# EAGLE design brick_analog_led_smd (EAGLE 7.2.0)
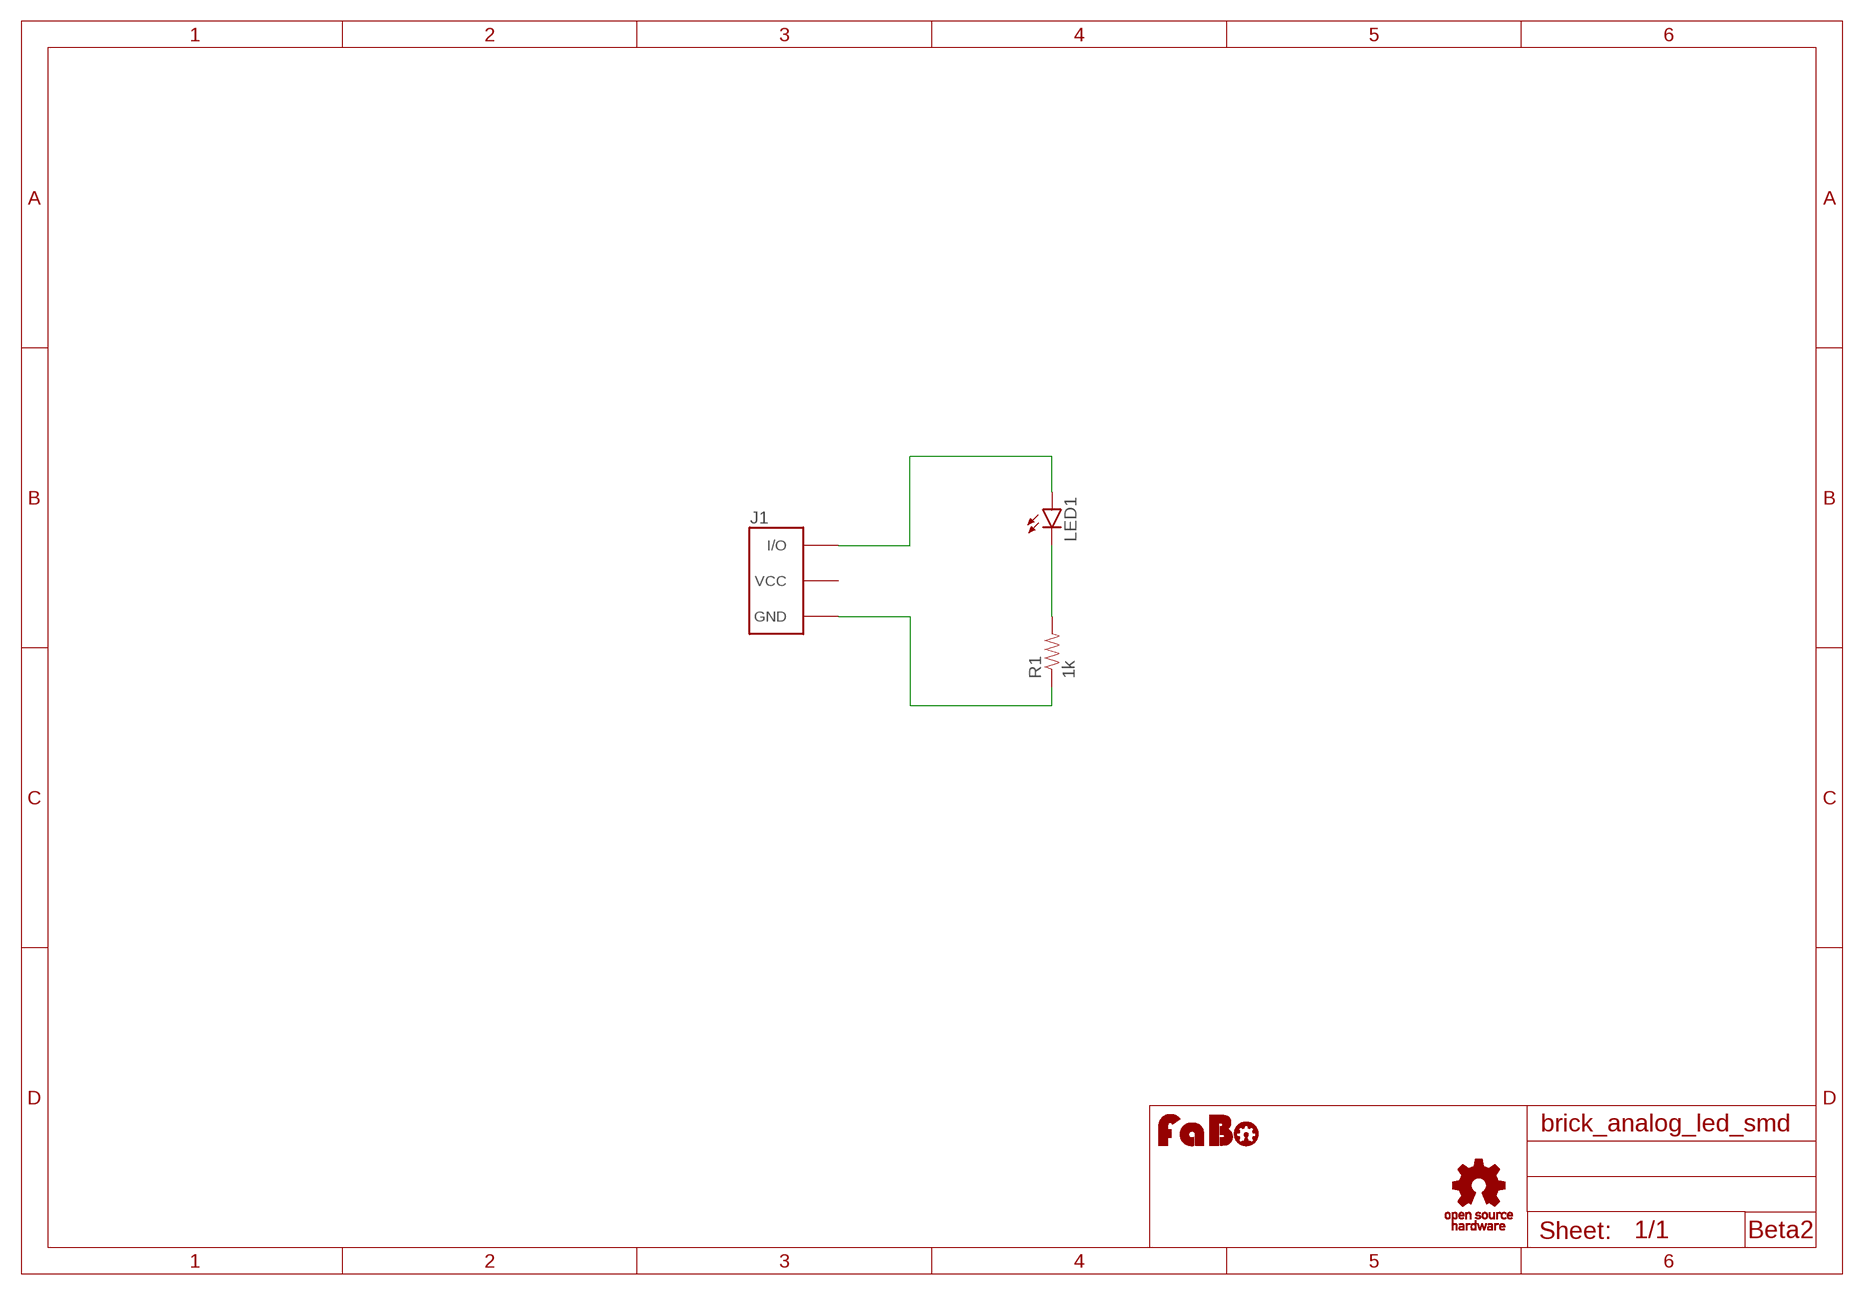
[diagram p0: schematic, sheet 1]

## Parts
J1  BRICK_3PIN  [BRICK_3PIN]
LED1  LED-EIA0603  [EIA0603-LED]
R1  1k  RES-EIA0603  [EIA0603]
U$2  LOGO_FABO-M  [LOGO_FABO_M]
U$4  LOGO_OSHW_T-M  [LOGO_OSHW_T_M]

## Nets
GND: J1.GND R1.1
N$1: J1.IN/OUT(I/O) LED1.A
N$3: LED1.C R1.2
Unconnected: J1.VCC

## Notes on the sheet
- Beta2

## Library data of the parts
J1 = Gclue:BRICK_3PIN: FaBo Brick 3pin
LED1 = Gclue:LED: LED
R1 = Gclue:RES
U$2 = FaBo:LOGO_FABO
U$4 = Gclue:LOGO_OSHW_T

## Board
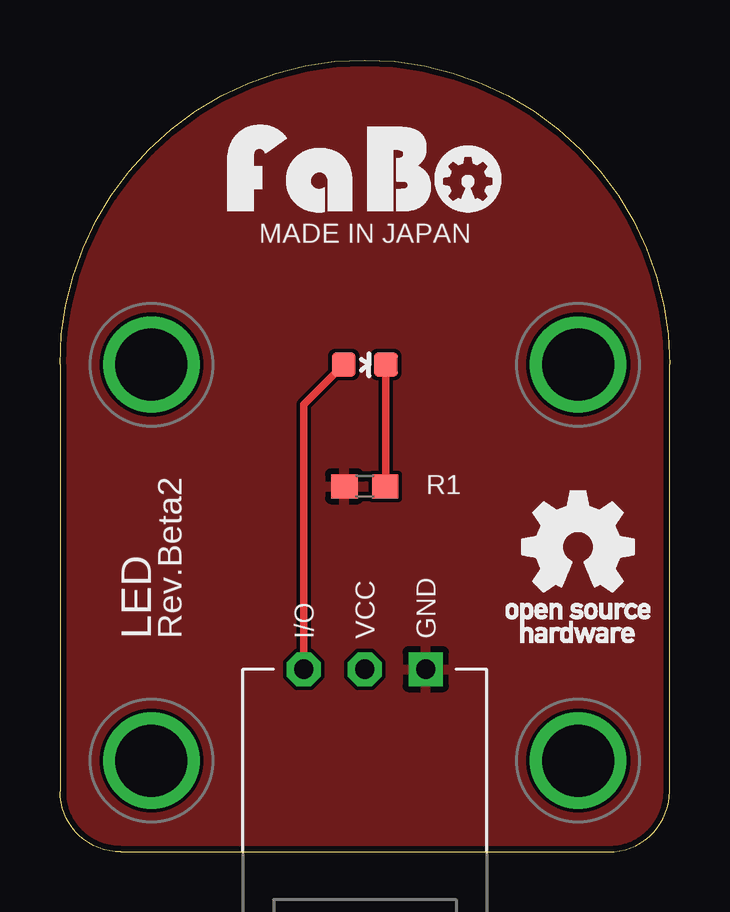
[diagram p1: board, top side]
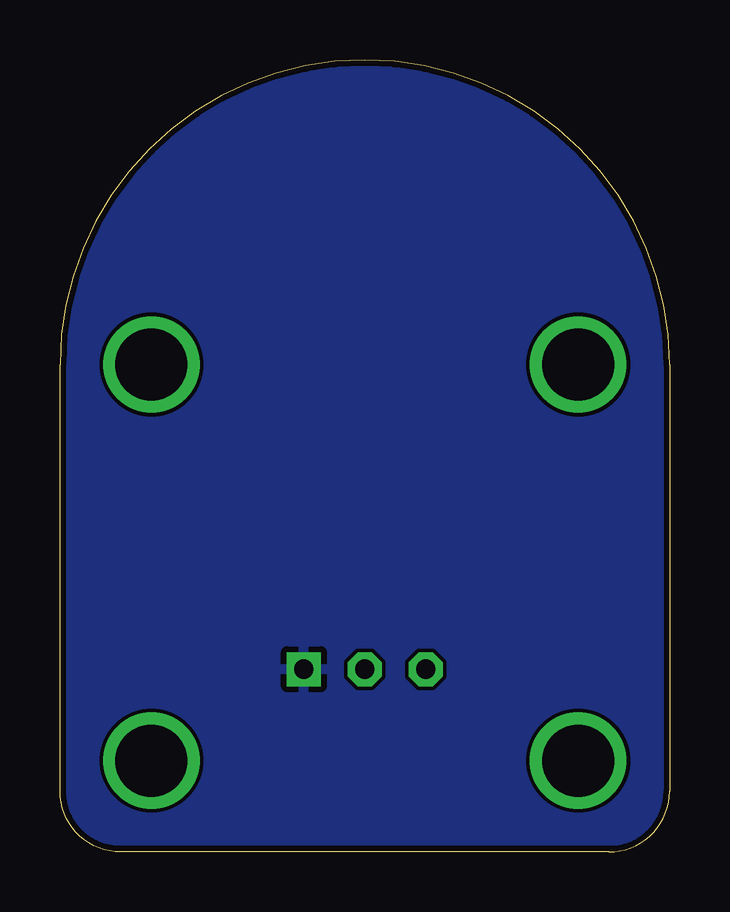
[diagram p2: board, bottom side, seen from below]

Size 25.4 x 33.02 mm. Coordinates in mm from the lower left corner, seen from the top.
Copper layers (1*16): Top 0.035mm / dielectric 1.5mm / Bottom 0.035mm
Design rules "Elecrow_2-layer_eagle_rule": minimum track width 6mil, minimum drill 12mil, track to track 6mil, track to pad 6mil, pad to pad 6mil, via to via 6mil, smd to smd 0mil, copper to edge 10mil, drill to drill 10mil, minimum pad ring 10mil, minimum via ring 6mil, stop-mask expansion 2mil, vias tented up to drill 100mil, thermal gap 10mil

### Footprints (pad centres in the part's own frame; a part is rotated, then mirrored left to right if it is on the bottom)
BRICK_3PIN = drill 0.8 pad 1.422 square: GND 2.54,-8.89 | drill 0.8 pad 1.422 octagon: IN/OUT -2.54,-8.89; VCC 0,-8.89 | drill 3 pad 3.81: P$5 -8.89,3.81; P$6 8.89,3.81; P$7 -8.89,-12.7; P$8 8.89,-12.7
EIA0603-LED = smd 1 x 1: A 0,-0.877; C 0,0.877
EIA0603 = smd 1.1 x 1: 1 -0.85,0; 2 0.85,0

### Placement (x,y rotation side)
J1  12.7,16.51 0 top
LED1  12.7,20.32 270 top
R1  12.7,15.24 0 top
U$2  12.7,26.67 0 top
U$4  21.59,12.7 0 top

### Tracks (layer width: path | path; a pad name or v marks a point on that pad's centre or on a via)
GND
  pour Bottom: -1.27,-1.27 26.67,-1.27 26.67,34.29 -1.27,34.29
  pour Top: -1.27,-1.27 26.67,-1.27 26.67,34.29 -1.27,34.29
N$1
  Top 0.305: J1.IN/OUT 10.16,18.66 LED1.A
N$3
  Top 0.305: LED1.C 13.58,15.27 R1.2

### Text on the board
tPlace: MADE IN JAPAN | LED | Rev.Beta2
